FUNCTION_BLOCK FB_SignalHandlingIntern //IMPLEMENTS I_SignalHandling
VAR_INPUT
	bInput				: BOOL;			// 输入信号
END_VAR
VAR_OUTPUT
	bOut				: BOOL;			// 输出信号
END_VAR
VAR
	bEnableLocal		: BOOL;			// 本地的输入变量
END_VAR

// =========================================================
;
// =========================================================

METHOD Enable
VAR_INPUT
	bEnable		: BOOL;
END_VAR
// =========================================================
// Store input in local variable

	bEnableLocal := bEnable;

// =========================================================
END_METHOD

METHOD SetOutput
VAR_INPUT
END_VAR
// =========================================================

bOut := bInput AND bEnableLocal;

// =========================================================
END_METHOD

END_FUNCTION_BLOCK
